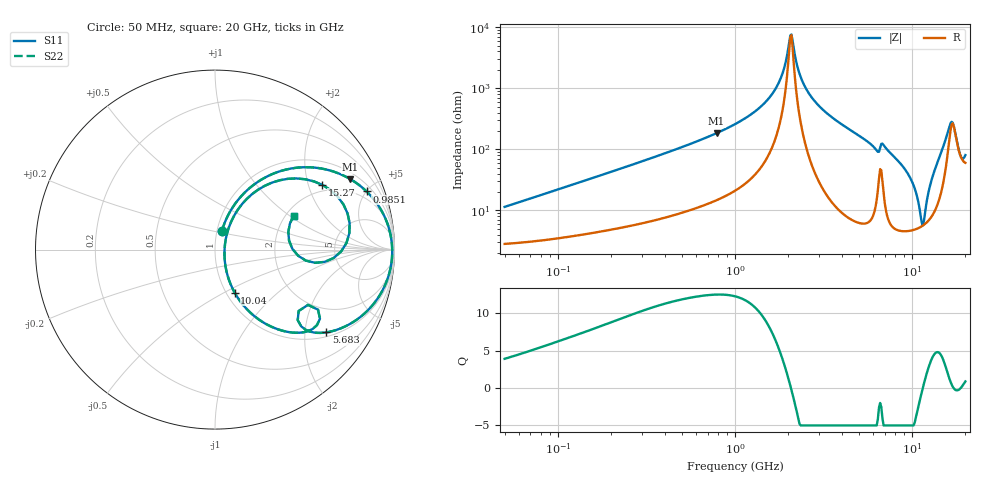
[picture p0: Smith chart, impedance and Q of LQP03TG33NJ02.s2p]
!Murata Part Number: LQP03TG33NJ02
!These Parameters are Measured in Series Mode Connection
!  o--[Z]--o
!Port1  Port2
!  o-------o
!Freq. Start=50[MHz] Stop=20[GHz], 401[Steps]
# Hz S RI R 50
!Freq.(Hz) S11(Real) S11(Imag) S21(Real) S21(Imag) S12(Real) S12(Imag) S22(Real) S22(Imag)
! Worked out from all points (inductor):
!   401 points, 50 MHz to 20 GHz, reference 50 ohm
!   read as one part in series: L = 34.9 nH near 51.52 MHz
!   highest Q = 12.5 at 786.9 MHz (marker M1), where L = 37.1 nH
!   self-resonance near 2.052 GHz
!   S11 on the Smith chart (normalised r, x): 50 MHz: 1.06, +0.22; 985.1 MHz: 1.41, +5.02; 5.683 GHz: 1.13, -2.59; 10.04 GHz: 1.09, -0.56; 15.27 GHz: 1.76, +2.48; 20 GHz: 2.20, +1.07
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5e7  0.0385 0.1032  0.9615 -0.1032  0.9615 -0.1032  0.0385 0.1032
1.364002e8  0.1091 0.2511  0.8909 -0.2511  0.8909 -0.2511  0.1091 0.2511
3.721004e8  0.3955 0.4459  0.6045 -0.4459  0.6045 -0.4459  0.3955 0.4459
7.868965e8  0.7545 0.3923  0.2455 -0.3923  0.2455 -0.3923  0.7545 0.3923
9.85133e8  0.8447 0.3239  0.1553 -0.3239  0.1553 -0.3239  0.8447 0.3239
1e9  0.85 0.3187  0.15 -0.3187  0.15 -0.3187  0.85 0.3187
1.639343e9  0.9709 0.1123  0.0291 -0.1123  0.0291 -0.1123  0.9709 0.1123
1.848039e9  0.9827 0.0554  0.0173 -0.0554  0.0173 -0.0554  0.9827 0.0554
2.05233e9  0.9872 0.00438  0.0128 -0.00438  0.0128 -0.00438  0.9872 0.00438
2.114743e9  0.9874 -0.0104  0.0126 0.0104  0.0126 0.0104  0.9874 -0.0104
2.348516e9  0.9844 -0.0627  0.0156 0.0627  0.0156 0.0627  0.9844 -0.0627
2.728004e9  0.9692 -0.1385  0.0308 0.1385  0.0308 0.1385  0.9692 -0.1385
5.683258e9  0.621 -0.461  0.379 0.461  0.379 0.461  0.621 -0.461
6.601595e9  0.518 -0.3079  0.482 0.3079  0.482 0.3079  0.518 -0.3079
7.442007e9  0.4519 -0.4634  0.5481 0.4634  0.5481 0.4634  0.4519 -0.4634
1.004137e10  0.1096 -0.2397  0.8904 0.2397  0.8904 0.2397  0.1096 -0.2397
1.149051e10  0.0532 -0.000407  0.9468 0.000407  0.9468 0.000407  0.0532 -0.000407
1.314879e10  0.1766 0.2821  0.8234 -0.2821  0.8234 -0.2821  0.1766 0.2821
1.527346e10  0.5985 0.3604  0.4015 -0.3604  0.4015 -0.3604  0.5985 0.3604
1.670968e10  0.7484 0.0906  0.2516 -0.0906  0.2516 -0.0906  0.7484 0.0906
1.774144e10  0.6107 -0.0686  0.3893 0.0686  0.3893 0.0686  0.6107 -0.0686
2e10  0.438 0.1879  0.562 -0.1879  0.562 -0.1879  0.438 0.1879
